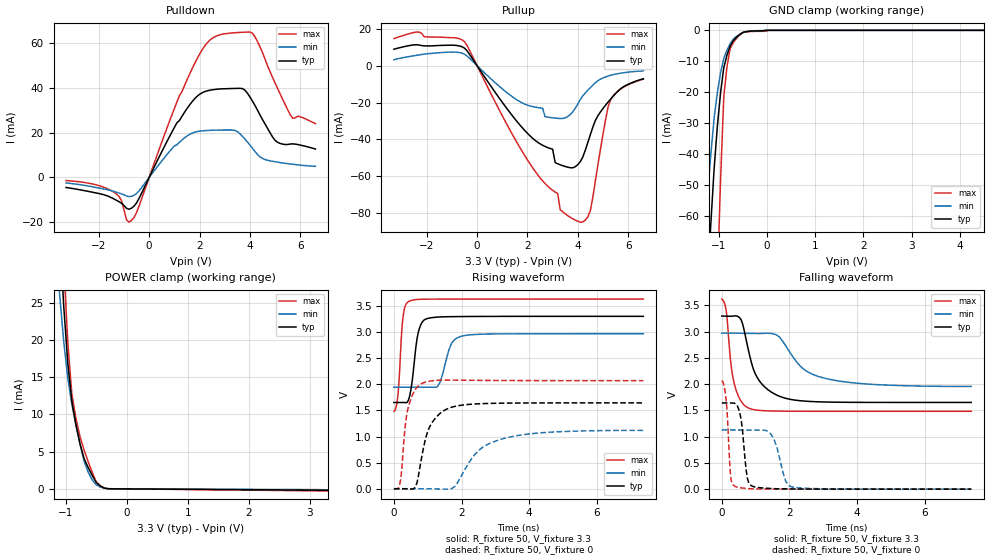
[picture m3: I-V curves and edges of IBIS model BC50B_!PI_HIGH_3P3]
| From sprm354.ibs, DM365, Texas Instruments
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|   Model Cell BC50B_!PI_HIGH_3P3
|BC1833DV50BTHYPBFZP_!PI_HIGH_3P3
[Model]   BC50B_!PI_HIGH_3P3
Model_type   I/O
Polarity   Non-Inverting
Enable   Active-Low
Vinl =  0.8V
Vinh =  2V
Cref =  15pF
Rref =  100.00M
Vref =  0V
Vmeas =  1.65
C_comp   1.614302p   1.431606p   1.718607p
[Model Spec]
Vinl   0.8V   0.8V   0.8V
Vinh   2V   2V   2V
[Temperature Range]   25   125   -40
[Voltage Range]   3.3   2.97   3.63
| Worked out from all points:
|   slope of the pulldown table from 0 to 0.495 V, typ, clamps not added: 43.6 ohm
|   slope of the pullup table from 0 to 0.495 V, typ, clamps not added: 49.2 ohm
|   GND clamp passes 1 mA (typ) near -0.53 V on its own axis
|   POWER clamp passes 1 mA (typ) near -0.51 V on its own axis
|   rising waveform, R_fixture 50, V_fixture 3.3: 20-80 % time 191ps typ, 274ps min, 121ps max; typ from 1.65 V to 3.3 V
|   rising waveform, R_fixture 50, V_fixture 0: 20-80 % time 436ps typ, 951ps min, 232ps max; typ from 0.004 V to 1.65 V
|   falling waveform, R_fixture 50, V_fixture 3.3: 20-80 % time 537ps typ, 945ps min, 248ps max; typ from 3.29 V to 1.65 V
|   falling waveform, R_fixture 50, V_fixture 0: 20-80 % time 154ps typ, 282ps min, 108ps max; typ from 1.64 V to 0.004 V
[POWER_clamp]
|   voltage   I(typ)   I(min)   I(max)
-3.3V     629.6mA    736.9mA    707.5mA
-1.1V     34.82mA    26.09mA    44.23mA
-1.033V   24.6mA     19.83mA    30.28mA
-966.7mV  16.93mA    14.92mA    19.78mA
-900mV    11.8mA     11.34mA    12.75mA
-833.3mV  8.649mA    8.605mA    9.544mA
-700mV    4.094mA    3.78mA     5.255mA
-633.3mV  2.89mA     2.285mA    3.679mA
-500mV    861.8uA    547.7uA    977.6uA
-433.3mV  388.5uA    262.3uA    416.9uA
-300mV    25.98uA    21.97uA    32.37uA
3.3V      -180.6uA   -153.3uA   -280.3uA
[Pulldown]
|   voltage   I(typ)   I(min)   I(max)
-3.3V     -4.448mA   -2.4mA     -1.374mA
-1.4V     -9.542mA   -6.187mA   -6.549mA
-900mV    -13.71mA   -8.202mA   -18.81mA
-700mV    -13.65mA   -8.389mA   -19.1mA
1.7V      33.68mA    19.73mA    48.3mA
2.3V      38.57mA    20.92mA    59.89mA
2.9V      39.49mA    21.13mA    63.8mA
3.7V      39.58mA    18.37mA    64.65mA
4.1V      34.01mA    13mA       64.27mA
5V        16.52mA    7.025mA    42.04mA
5.7V      14.97mA    5.897mA    26.31mA
6.6V      12.66mA    4.964mA    23.97mA
[Pullup]
|   voltage   I(typ)   I(min)   I(max)
-3.3V     8.925mA    3.225mA    14.72mA
-500mV    9.531mA    6.242mA    13.04mA
1.6V      -30.57mA   -18.73mA   -42.11mA
2.7V      -43.89mA   -27.7mA    -64.03mA
3V        -45.38mA   -28.31mA   -67.67mA
3.2V      -53.28mA   -28.6mA    -69.43mA
3.3V      -53.83mA   -28.7mA    -78.25mA
4.1V      -52.1mA    -18.35mA   -84.99mA
4.5V      -37.33mA   -11.85mA   -78.49mA
5.1V      -21.45mA   -6.119mA   -29.35mA
5.3V      -18.16mA   -5.226mA   -18.53mA
6.6V      -7.127mA   -2.839mA   -7.361mA
[GND_clamp]
|   voltage   I(typ)   I(min)   I(max)
-3.3V     -715.9mA   -742.1mA   -1.572A
-1.3V     -98.68mA   -65.29mA   -247.1mA
-1.233V   -79.85mA   -52.03mA   -203.2mA
-1.167V   -61.82mA   -39.7mA    -160.2mA
-1.1V     -44.6mA    -28.28mA   -118mA
-1.033V   -30.94mA   -20.09mA   -80.41mA
-966.7mV  -20.1mA    -13.69mA   -48.21mA
-900mV    -12.08mA   -9.068mA   -21.4mA
-833.3mV  -7.953mA   -6.384mA   -11.68mA
-766.7mV  -5.031mA   -4.295mA   -5.845mA
-500mV    -657.6uA   -656.9uA   -717uA
6.6V      0A         0A         0A
[Ramp]
| variable   typ   min   max
dV/dt_f  0.9886301/0.5346872n  0.6149409/0.9836446n   1.287534/0.2471897n
dV/dt_r  0.9894115/0.4355294n  0.6802764/0.9803182n   1.249415/0.2354323n
R_load = 50
[Rising Waveform]
R_fixture = 50
V_fixture = 3.3
V_fixture_min = 2.97
V_fixture_max = 3.63
|   time   V(typ)   V(min)   V(max)
0s        1.652V     1.945V     1.483V
120ps     1.652V     1.945V     1.802V
276ps     1.652V     1.945V     3.317V
468ps     1.783V     1.945V     3.593V
720ps     2.991V     1.945V     3.624V
978ps     3.256V     1.945V     3.628V
1.278ns   3.284V     1.947V     3.629V
1.71ns    3.294V     2.792V     3.629V
2.058ns   3.296V     2.928V     3.63V
7.374ns   3.3V       2.968V     3.63V
[Rising Waveform]
R_fixture = 50
V_fixture = 0
V_fixture_min = 0
V_fixture_max = 0
|   time   V(typ)   V(min)   V(max)
0s        4.157mV    2.533mV    2.402mV
198ps     4.16mV     2.536mV    175.3mV
432ps     -2.275mV   2.531mV    1.576V
648ps     55.39mV    2.524mV    1.917V
870ps     773.5mV    2.524mV    2.029V
1.194ns   1.327V     2.137mV    2.072V
1.8ns     1.578V     46.94mV    2.08V
2.406ns   1.624V     668.8mV    2.076V
3.108ns   1.639V     938mV      2.073V
7.374ns   1.645V     1.119V     2.07V
[Falling Waveform]
R_fixture = 50
V_fixture = 3.3
V_fixture_min = 2.97
V_fixture_max = 3.63
|   time   V(typ)   V(min)   V(max)
0s        3.295V     2.97V      3.618V
120ps     3.292V     2.97V      3.436V
276ps     3.291V     2.97V      2.351V
372ps     3.298V     2.97V      2V
576ps     3.216V     2.968V     1.669V
792ps     2.629V     2.965V     1.545V
1.158ns   2.022V     2.964V     1.499V
1.974ns   1.718V     2.641V     1.485V
3.294ns   1.658V     2.077V     1.484V
7.374ns   1.652V     1.957V     1.484V
[Falling Waveform]
R_fixture = 50
V_fixture = 0
V_fixture_min = 0
V_fixture_max = 0
|   time   V(typ)   V(min)   V(max)
0s        1.642V     1.129V     2.071V
138ps     1.642V     1.129V     1.623V
276ps     1.642V     1.129V     176mV
408ps     1.626V     1.128V     51.56mV
576ps     1.305V     1.128V     28.28mV
756ps     209.8mV    1.127V     15.47mV
906ps     59.32mV    1.127V     10.31mV
1.452ns   16.03mV    1.05V      6.23mV
2.058ns   7.256mV    48.81mV    5.95mV
7.374ns   4.165mV    3.561mV    5.925mV
